| IBIS file stm32h523_533_ufbga144.ibs
[IBIS ver] 4.2
[File name] stm32h523_533_ufbga144.ibs
[File Rev] 0.2
[Date] 07-05-2024
[Source] Data Created at STMicroelectronics
[Notes]  File originated from ELDO simulations.
[Disclaimer]  This information is for modeling purpose only and is
   not guaranteed. The information is subject to change without
   notice.
[Copyright] Copyright 2024 STMicroelectronics Inc.
|   Component stm32h523_533_ufbga144
[Component] stm32h523_533_ufbga144
[Manufacturer] STMicroelectronics
[Package]
| variable   typ   min   max
R_pkg  0  NA  NA
L_pkg  0  NA  NA
C_pkg  0  NA  NA
[Pin]   signal_name   model_name
A1  VSS  gnd
A2  PB9  io8_ft_i3c_spi
A3  PB7  io8_ft_i3c_spi
A4  PB4  io8_ft_i3c_spi
A5  PG15  io8_ft_i3c_spi
A6  PG12  io8_ft_i3c_spi
A7  PG11  io8_ft_i3c_spi
A8  PD7  io8_ft_i3c_spi
A9  PD4  io8_ft_i3c_spi
A10  PD2  io8_ft_i3c_spi
A11  PC10  io8_ft_i3c_spi
A12  VSS  gnd
B1  PE2  io8_ft_i3c_spi
B2  PE0  io8_ft_i3c_spi
B3  PB8  io8_ft_i3c_spi
B4  PB6  io8_ft_i3c_spi
B5  PB3  io8_ft_i3c_spi
B6  PG14  io8_ft_i3c_spi
B7  PG10  io8_ft_i3c_spi
B8  PD6  io8_ft_i3c_spi
B9  PD3  io8_ft_i3c_spi
B10  PC12  io8_ft_i3c_spi
B11  PA14  io8_ft_i3c_spi
B12  PA10  io8_ft_i3c_spi
C1  VBAT  power
C2  PE4  io8_ft_i3c_spi
C3  PE3  io8_ft_i3c_spi
C4  BOOT0  vpphv
C5  VDDIO2  power
C6  VSS  gnd
C7  VDDIO2  power
C8  PD5  io8_ft_i3c_spi
C9  PD1  io8_ft_i3c_spi
C10  VDDUSB  power
C11  PA12  io8usb_ft_i3c_spi_phy
C12  PA11  io8usb_ft_i3c_spi_phy
D1  PC15-OSC32_OUT  io_ft_tamp
D2  PC14-OSC32_IN  io_ft_tamp
D3  PE5  io8_ft_i3c_spi
D4  VSS  gnd
D5  VCAP  nc
D6  PG13  io8_ft_i3c_spi
D7  PG9  io8_ft_i3c_spi
D8  PD0  io8_ft_i3c_spi
D9  PC11  io8_ft_i3c_spi
D10  VSS  gnd
D11  PA9  io8_ft_i3c_spi
D12  PA8  io8_ft_i3c_spi
E1  PF1  io8_ft_i3c_spi
E2  PF0  io8_ft_i3c_spi
E3  PC13  io8_ft_i3c_spi_v33
E4  PE6  io8_ft_i3c_spi
E5  VDD  power
E6  PB5  io8_ft_i3c_spi
E7  VDD  power
E8  PA15  io8_ft_i3c_spi
E9  PA13  io8_ft_i3c_spi
E10  PC9  io8_ft_i3c_spi
E11  PC8  io8_ft_i3c_spi
E12  PC7  io8_ft_i3c_spi
F1  PF5  io8_ft_i3c_spi
F2  PF4  io8_ft_i3c_spi
F3  PF3  io8_ft_i3c_spi
F4  PF2  io8_ft_i3c_spi
F5  VSS  gnd
F6  VDD  power
F7  VSS  gnd
F8  VDD  power
F9  PC6  io8_ft_i3c_spi
F10  PG8  io8_ft_i3c_spi
F11  PG7  io8_ft_i3c_spi
F12  PG6  io8_ft_i3c_spi
G1  PF6  io8_ft_i3c_spi
G2  PF7  io8_ft_i3c_spi
G3  PF9  io8_ft_i3c_spi
G4  PF8  io8_ft_i3c_spi
G5  VDD  power
G6  VSS  gnd
G7  VDD  power
G8  PD11  io8_ft_i3c_spi
G9  PD15  io8_ft_i3c_spi
G10  PG3  io8_ft_i3c_spi
G11  PG4  io8_ft_i3c_spi
G12  PG5  io8_ft_i3c_spi
H1  PH0-OSC_IN  io8_ft_i3c_spi
H2  PH1-OSC_OUT  io8_ft_i3c_spi
H3  PF10  io8_ft_i3c_spi
H4  VREFM  nc
H5  VSS  gnd
H6  VDD  power
H7  VSS  gnd
H8  PB14  nc
H9  PB15  io8_ft_spi
H10  PD12  io8_ft_i3c_spi
H11  PD14  io8_ft_i3c_spi
H12  PG2  io8_ft_i3c_spi
J1  NRST  ioreset_ft_v33
J2  PC0  io8_ft_spi
J3  VREFP  nc
J4  VDDA  nc
J5  PA7  io8_ft_spi
J6  PB1  io8_ft_spi
J7  PG1  io8_ft_i3c_spi
J8  VCAP  nc
J9  VSS  gnd
J10  PD8  io8_ft_i3c_spi
J11  PD9  io8_ft_i3c_spi
J12  PD13  io8_ft_i3c_spi
K1  PC2  io8_ft_spi
K2  PC1  io8_ft_spi
K3  VSSA  nc
K4  PA2  io8_ft_spi
K5  PC4  io8_ft_spi
K6  PB2  io8_ft_i3c_spi
K7  PF15  io8_ft_i3c_spi
K8  PE9  io8_ft_i3c_spi
K9  PE12  io8_ft_i3c_spi
K10  PE15  io8_ft_i3c_spi
K11  PB13  nc
K12  PD10  io8_ft_i3c_spi
L1  PC3  io8_ft_spi
L2  PA0  io8_ft_spi
L3  PA1  io8_ft_spi_tamp
L4  PA5  io8_ft_spi
L5  PC5  io8_ft_spi
L6  PF11  io8_ft_spi
L7  PF14  io8_ft_spi
L8  PE7  io8_ft_i3c_spi
L9  PE10  io8_ft_i3c_spi
L10  PE14  io8_ft_i3c_spi
L11  PB10  io8_ft_i3c_spi
L12  PB12  io8_ft_i3c_spi
M1  VSS  gnd
M2  PA3  io8_ft_spi
M3  PA4  io8_ft_spi
M4  PA6  io8_ft_spi
M5  PB0  io8_ft_spi
M6  PF12  io8_ft_spi
M7  PF13  io8_ft_spi
M8  PG0  io8_ft_i3c_spi
M9  PE8  io8_ft_i3c_spi
M10  PE11  io8_ft_i3c_spi
M11  PE13  io8_ft_i3c_spi
M12  VSS  gnd
[Package Model]   478-ufbga10x10-144-240126
[Pin Mapping]   pulldown_ref   pullup_ref   | Comment
A1  gndio  nc
A2  gndio  vddmmc
A3  gndio  vddio
A4  gndio  vddio
A5  gndio  vddio
A6  gndio  vddmmc
A7  gndio  vddmmc
A8  gndio  vddmmc
A9  gndio  vddio
A10  gndio  vddio
A11  gndio  vddio
A12  gndio  nc
B1  gndio  vddio
B2  gndio  vddio
B3  gndio  vddmmc
B4  gndio  vddio
B5  gndio  vddio
B6  gndio  vddmmc
B7  gndio  vddmmc
B8  gndio  vddmmc
B9  gndio  vddio
B10  gndio  vddio
B11  gndio  vddio
B12  gndio  vddio
C1  nc  vsw
C2  gndio  vddio
C3  gndio  vddio
C4  gndio  vddio
C5  nc  vddmmc
C6  gndio  nc
C7  nc  vddmmc
C8  gndio  vddio
C9  gndio  vddio
C10  nc  vddusb
C11  gndio  vddusb  | Depending on IO usage
| C11  gndio  vddio  | Depending on IO usage
C12  gndio  vddusb  | Depending on IO usage
| C12  gndio  vddio  | Depending on IO usage
D1  gndio  vddio  | Depending on IO usage
| D1  gndio  vsw  | Depending on IO usage
D2  gndio  vddio  | Depending on IO usage
| D2  gndio  vsw  | Depending on IO usage
D3  gndio  vddio
D4  gndio  nc
D5  nc  nc
D6  gndio  vddmmc
D7  gndio  vddmmc
D8  gndio  vddio
D9  gndio  vddio
D10  gndio  nc
D11  gndio  vddio
D12  gndio  vddio
E1  gndio  vddio
E2  gndio  vddio
E3  gndio  vddio  | Depending on IO usage
| E3  gndio  vsw  | Depending on IO usage
E4  gndio  vddio
E5  nc  vddio
E6  gndio  vddio
E7  nc  vddio
E8  gndio  vddio
E9  gndio  vddio
E10  gndio  vddio
E11  gndio  vddio
E12  gndio  vddio
F1  gndio  vddio
F2  gndio  vddio
F3  gndio  vddio
F4  gndio  vddio
F5  gndio  nc
F6  nc  vddio
F7  gndio  nc
F8  nc  vddio
F9  gndio  vddio
F10  gndio  vddio
F11  gndio  vddio
F12  gndio  vddio
G1  gndio  vddio
G2  gndio  vddio
G3  gndio  vddio
G4  gndio  vddio
G5  nc  vddio
G6  gndio  nc
G7  nc  vddio
G8  gndio  vddio
G9  gndio  vddio
G10  gndio  vddio
G11  gndio  vddio
G12  gndio  vddio
H1  gndio  vddio
H2  gndio  vddio
H3  gndio  vddio
H4  nc  nc
H5  gndio  nc
H6  nc  vddio
H7  gndio  nc
H8  nc  nc
H9  gndio  vddio
H10  gndio  vddio
H11  gndio  vddio
H12  gndio  vddio
J1  gndio  vddio
J2  gndio  vddio
J3  nc  nc
J4  nc  nc
J5  gndio  vddio
J6  gndio  vddio
J7  gndio  vddio
J8  nc  nc
J9  gndio  nc
J10  gndio  vddio
J11  gndio  vddio
J12  gndio  vddio
K1  gndio  vddio
K2  gndio  vddio
K3  nc  nc
K4  gndio  vddio
K5  gndio  vddio
K6  gndio  vddio
K7  gndio  vddio
K8  gndio  vddio
K9  gndio  vddio
K10  gndio  vddio
K11  nc  nc
K12  gndio  vddio
L1  gndio  vddio
L2  gndio  vddio
L3  gndio  vddio
L4  gndio  vddio
L5  gndio  vddio
L6  gndio  vddio
L7  gndio  vddio
L8  gndio  vddio
L9  gndio  vddio
L10  gndio  vddio
L11  gndio  vddio
L12  gndio  vddio
M1  gndio  nc
M2  gndio  vddio
M3  gndio  vddio
M4  gndio  vddio
M5  gndio  vddio
M6  gndio  vddio
M7  gndio  vddio
M8  gndio  vddio
M9  gndio  vddio
M10  gndio  vddio
M11  gndio  vddio
M12  gndio  nc
|[Diff Pin]  inv_pin  vdiff  tdelay_typ  tdelay_min  tdelay_max
|C11  C12  NA  NA  NA  NA
[Model Selector] io8_ft_i3c_spi
io8_ft_spi_ls_1v2 "GPIO SPI - 5V tolerant - low speed - 1.2V range"
io8_ft_spi_ls_1v8 "GPIO SPI - 5V tolerant - low speed - 1.8V range"
io8_ft_spi_ls_3v3 "GPIO SPI - 5V tolerant - low speed - 3.3V range"
io8_ft_spi_ms_1v2 "GPIO SPI - 5V tolerant - med speed - 1.2V range"
io8_ft_spi_ms_1v8 "GPIO SPI - 5V tolerant - med speed - 1.8V range"
io8_ft_spi_ms_3v3 "GPIO SPI - 5V tolerant - med speed - 3.3V range"
io8_ft_spi_fs_1v2 "GPIO SPI - 5V tolerant - fast speed - 1.2V range"
io8_ft_spi_fs_1v8 "GPIO SPI - 5V tolerant - fast speed - 1.8V range"
io8_ft_spi_fs_3v3 "GPIO SPI - 5V tolerant - fast speed - 3.3V range"
io8_ft_spi_hs_1v2 "GPIO SPI - 5V tolerant - high speed - 1.2V range"
io8_ft_spi_hs_1v8 "GPIO SPI - 5V tolerant - high speed - 1.8V range"
io8_ft_spi_hs_3v3 "GPIO SPI - 5V tolerant - high speed - 3.3V range"
io8_ft_hslv_spi_ls_1v2 "GPIO SPI low volt opt - 5V tolerant - low speed - 1.2V range"
io8_ft_hslv_spi_ls_1v8 "GPIO SPI low volt opt - 5V tolerant - low speed - 1.8V range"
io8_ft_hslv_spi_ls_2v5 "GPIO SPI low volt opt - 5V tolerant - low speed - 2.5V range"
io8_ft_hslv_spi_ms_1v2 "GPIO SPI low volt opt - 5V tolerant - med speed - 1.2V range"
io8_ft_hslv_spi_ms_1v8 "GPIO SPI low volt opt - 5V tolerant - med speed - 1.8V range"
io8_ft_hslv_spi_ms_2v5 "GPIO SPI low volt opt - 5V tolerant - med speed - 2.5V range"
io8_ft_hslv_spi_fs_1v2 "GPIO SPI low volt opt - 5V tolerant - fast speed - 1.2V range"
io8_ft_hslv_spi_fs_1v8 "GPIO SPI low volt opt - 5V tolerant - fast speed - 1.8V range"
io8_ft_hslv_spi_fs_2v5 "GPIO SPI low volt opt - 5V tolerant - fast speed - 2.5V range"
io8_ft_hslv_spi_hs_1v2 "GPIO SPI low volt opt - 5V tolerant - high speed - 1.2V range"
io8_ft_hslv_spi_hs_1v8 "GPIO SPI low volt opt - 5V tolerant - high speed - 1.8V range"
io8_ft_hslv_spi_hs_2v5 "GPIO SPI low volt opt - 5V tolerant - high speed - 2.5V range"
io8_ft_i3c_spi_ls_1v2 "GPIO SPI with I3C open-drain - 5V tolerant - low speed - 1.2V range"
io8_ft_i3c_spi_ls_1v8 "GPIO SPI with I3C open-drain - 5V tolerant - low speed - 1.8V range"
io8_ft_i3c_spi_ls_3v3 "GPIO SPI with I3C open-drain - 5V tolerant - low speed - 3.3V range"
io8_ft_i3c_spi_ms_1v2 "GPIO SPI with I3C open-drain - 5V tolerant - med speed - 1.2V range"
io8_ft_i3c_spi_ms_1v8 "GPIO SPI with I3C open-drain - 5V tolerant - med speed - 1.8V range"
io8_ft_i3c_spi_ms_3v3 "GPIO SPI with I3C open-drain - 5V tolerant - med speed - 3.3V range"
io8_ft_i3c_spi_fs_1v2 "GPIO SPI with I3C open-drain - 5V tolerant - fast speed - 1.2V range"
io8_ft_i3c_spi_fs_1v8 "GPIO SPI with I3C open-drain - 5V tolerant - fast speed - 1.8V range"
io8_ft_i3c_spi_fs_3v3 "GPIO SPI with I3C open-drain - 5V tolerant - fast speed - 3.3V range"
io8_ft_i3c_spi_hs_1v2 "GPIO SPI with I3C open-drain - 5V tolerant - high speed - 1.2V range"
io8_ft_i3c_spi_hs_1v8 "GPIO SPI with I3C open-drain - 5V tolerant - high speed - 1.8V range"
io8_ft_i3c_spi_hs_3v3 "GPIO SPI with I3C open-drain - 5V tolerant - high speed - 3.3V range"
io8_ft_hslv_i3c_spi_ls_1v2 "GPIO SPI low volt opt with I3C open-drain - 5V tolerant - low speed - 1.2V range"
io8_ft_hslv_i3c_spi_ls_1v8 "GPIO SPI low volt opt with I3C open-drain - 5V tolerant - low speed - 1.8V range"
io8_ft_hslv_i3c_spi_ls_2v5 "GPIO SPI low volt opt with I3C open-drain - 5V tolerant - low speed - 2.5V range"
io8_ft_hslv_i3c_spi_ms_1v2 "GPIO SPI low volt opt with I3C open-drain - 5V tolerant - med speed - 1.2V range"
io8_ft_hslv_i3c_spi_ms_1v8 "GPIO SPI low volt opt with I3C open-drain - 5V tolerant - med speed - 1.8V range"
io8_ft_hslv_i3c_spi_ms_2v5 "GPIO SPI low volt opt with I3C open-drain - 5V tolerant - med speed - 2.5V range"
io8_ft_hslv_i3c_spi_fs_1v2 "GPIO SPI low volt opt with I3C open-drain - 5V tolerant - fast speed - 1.2V range"
io8_ft_hslv_i3c_spi_fs_1v8 "GPIO SPI low volt opt with I3C open-drain - 5V tolerant - fast speed - 1.8V range"
io8_ft_hslv_i3c_spi_fs_2v5 "GPIO SPI low volt opt with I3C open-drain - 5V tolerant - fast speed - 2.5V range"
io8_ft_hslv_i3c_spi_hs_1v2 "GPIO SPI low volt opt with I3C open-drain - 5V tolerant - high speed - 1.2V range"
io8_ft_hslv_i3c_spi_hs_1v8 "GPIO SPI low volt opt with I3C open-drain - 5V tolerant - high speed - 1.8V range"
io8_ft_hslv_i3c_spi_hs_2v5 "GPIO SPI low volt opt with I3C open-drain - 5V tolerant - high speed - 2.5V range"
io8_ft_i3c_fmp_spi_3v3 "GPIO SPI with I3C fm+ open-drain - 5V tolerant - 3.3V range"
io8_ft_i3c_fmp_spi_1v8 "GPIO SPI with I3C fm+ open-drain - 5V tolerant - 1.8V range"
io8_ft_i3c_fmp_spi_1v2 "GPIO SPI with I3C fm+ open-drain - 5V tolerant - 1.2V range"
[Model Selector] io8_ft_i3c_spi_v33
io8_ft_spi_v33_ls_1v2 ""GPIO SPI V33 - 5V tolerant - low speed - 1.2V range"
io8_ft_spi_v33_ls_1v8 ""GPIO SPI V33 - 5V tolerant - low speed - 1.8V range"
io8_ft_spi_v33_ls_3v3 ""GPIO SPI V33 - 5V tolerant - low speed - 3.3V range"
io8_ft_spi_v33_ms_1v2 ""GPIO SPI V33 - 5V tolerant - med speed - 1.2V range"
io8_ft_spi_v33_ms_1v8 ""GPIO SPI V33 - 5V tolerant - med speed - 1.8V range"
io8_ft_spi_v33_ms_3v3 ""GPIO SPI V33 - 5V tolerant - med speed - 3.3V range"
io8_ft_spi_v33_fs_1v2 ""GPIO SPI V33 - 5V tolerant - fast speed - 1.2V range
io8_ft_spi_v33_fs_1v8 ""GPIO SPI V33 - 5V tolerant - fast speed - 1.8V range
io8_ft_spi_v33_fs_3v3 ""GPIO SPI V33 - 5V tolerant - fast speed - 3.3V range
io8_ft_spi_v33_hs_1v2 ""GPIO SPI V33 - 5V tolerant - high speed - 1.2V range
io8_ft_spi_v33_hs_1v8 ""GPIO SPI V33 - 5V tolerant - high speed - 1.8V range
io8_ft_spi_v33_hs_3v3 ""GPIO SPI V33 - 5V tolerant - high speed - 3.3V range
io8_ft_hslv_spi_v33_ls_1v2 "GPIO SPI V33 low volt opt - 5V tolerant - low speed - 1.2V range""
io8_ft_hslv_spi_v33_ls_1v8 "GPIO SPI V33 low volt opt - 5V tolerant - low speed - 1.8V range""
io8_ft_hslv_spi_v33_ls_2v5 "GPIO SPI V33 low volt opt - 5V tolerant - low speed - 2.5V range""
io8_ft_hslv_spi_v33_ms_1v2 "GPIO SPI V33 low volt opt - 5V tolerant - med speed - 1.2V range""
io8_ft_hslv_spi_v33_ms_1v8 "GPIO SPI V33 low volt opt - 5V tolerant - med speed - 1.8V range""
io8_ft_hslv_spi_v33_ms_2v5 "GPIO SPI V33 low volt opt - 5V tolerant - med speed - 2.5V range""
io8_ft_hslv_spi_v33_fs_1v2 "GPIO SPI V33 low volt opt - 5V tolerant - fast speed - 1.2V range"
io8_ft_hslv_spi_v33_fs_1v8 "GPIO SPI V33 low volt opt - 5V tolerant - fast speed - 1.8V range"
io8_ft_hslv_spi_v33_fs_2v5 "GPIO SPI V33 low volt opt - 5V tolerant - fast speed - 2.5V range"
io8_ft_hslv_spi_v33_hs_1v2 "GPIO SPI V33 low volt opt - 5V tolerant - high speed - 1.2V range"
io8_ft_hslv_spi_v33_hs_1v8 "GPIO SPI V33 low volt opt - 5V tolerant - high speed - 1.8V range"
io8_ft_hslv_spi_v33_hs_2v5 "GPIO SPI V33 low volt opt - 5V tolerant - high speed - 2.5V range"
io8_ft_i3c_spi_v33_ls_1v2 "GPIO SPI V33 with I3C open-drain - 5V tolerant - low speed - 1.2V range"
io8_ft_i3c_spi_v33_ls_1v8 "GPIO SPI V33 with I3C open-drain - 5V tolerant - low speed - 1.8V range"
io8_ft_i3c_spi_v33_ls_3v3 "GPIO SPI V33 with I3C open-drain - 5V tolerant - low speed - 3.3V range"
io8_ft_i3c_spi_v33_ms_1v2 "GPIO SPI V33 with I3C open-drain - 5V tolerant - med speed - 1.2V range"
io8_ft_i3c_spi_v33_ms_1v8 "GPIO SPI V33 with I3C open-drain - 5V tolerant - med speed - 1.8V range"
io8_ft_i3c_spi_v33_ms_3v3 "GPIO SPI V33 with I3C open-drain - 5V tolerant - med speed - 3.3V range"
io8_ft_i3c_spi_v33_fs_1v2 "GPIO SPI V33 with I3C open-drain - 5V tolerant - fast speed - 1.2V range"
io8_ft_i3c_spi_v33_fs_1v8 "GPIO SPI V33 with I3C open-drain - 5V tolerant - fast speed - 1.8V range"
io8_ft_i3c_spi_v33_fs_3v3 "GPIO SPI V33 with I3C open-drain - 5V tolerant - fast speed - 3.3V range"
io8_ft_i3c_spi_v33_hs_1v2 "GPIO SPI V33 with I3C open-drain - 5V tolerant - high speed - 1.2V range"
io8_ft_i3c_spi_v33_hs_1v8 "GPIO SPI V33 with I3C open-drain - 5V tolerant - high speed - 1.8V range"
io8_ft_i3c_spi_v33_hs_3v3 "GPIO SPI V33 with I3C open-drain - 5V tolerant - high speed - 3.3V range"
io8_ft_hslv_i3c_spi_v33_ls_1v2 "GPIO SPI V33 low volt opt with I3C open-drain - 5V tolerant - low speed - 1.2V range"
io8_ft_hslv_i3c_spi_v33_ls_1v8 "GPIO SPI V33 low volt opt with I3C open-drain - 5V tolerant - low speed - 1.8V range"
io8_ft_hslv_i3c_spi_v33_ls_2v5 "GPIO SPI V33 low volt opt with I3C open-drain - 5V tolerant - low speed - 2.5V range"
io8_ft_hslv_i3c_spi_v33_ms_1v2 "GPIO SPI V33 low volt opt with I3C open-drain - 5V tolerant - med speed - 1.2V range"
io8_ft_hslv_i3c_spi_v33_ms_1v8 "GPIO SPI V33 low volt opt with I3C open-drain - 5V tolerant - med speed - 1.8V range"
io8_ft_hslv_i3c_spi_v33_ms_2v5 "GPIO SPI V33 low volt opt with I3C open-drain - 5V tolerant - med speed - 2.5V range"
io8_ft_hslv_i3c_spi_v33_fs_1v2 "GPIO SPI V33 low volt opt with I3C open-drain - 5V tolerant - fast speed - 1.2V range"
io8_ft_hslv_i3c_spi_v33_fs_1v8 "GPIO SPI V33 low volt opt with I3C open-drain - 5V tolerant - fast speed - 1.8V range"
io8_ft_hslv_i3c_spi_v33_fs_2v5 "GPIO SPI V33 low volt opt with I3C open-drain - 5V tolerant - fast speed - 2.5V range"
io8_ft_hslv_i3c_spi_v33_hs_1v2 "GPIO SPI V33 low volt opt with I3C open-drain - 5V tolerant - high speed - 1.2V range"
io8_ft_hslv_i3c_spi_v33_hs_1v8 "GPIO SPI V33 low volt opt with I3C open-drain - 5V tolerant - high speed - 1.8V range"
io8_ft_hslv_i3c_spi_v33_hs_2v5 "GPIO SPI V33 low volt opt with I3C open-drain - 5V tolerant - high speed - 2.5V range"
io8_ft_i3c_fmp_spi_v33_3v3 "GPIO SPI V33 with I3C fm+ open-drain - 5V tolerant - 3.3V range"
io8_ft_i3c_fmp_spi_v33_1v8 "GPIO SPI V33 with I3C fm+ open-drain - 5V tolerant - 1.8V range"
io8_ft_i3c_fmp_spi_v33_1v2 "GPIO SPI V33 with I3C fm+ open-drain - 5V tolerant - 1.2V range"
[Model Selector] io8_ft_spi
io8_ft_spi_ls_1v2 "GPIO SPI - 5V tolerant - low speed - 1.2V range"
io8_ft_spi_ls_1v8 "GPIO SPI - 5V tolerant - low speed - 1.8V range"
io8_ft_spi_ls_3v3 "GPIO SPI - 5V tolerant - low speed - 3.3V range"
io8_ft_spi_ms_1v2 "GPIO SPI- 5V tolerant - med speed - 1.2V range"
io8_ft_spi_ms_1v8 "GPIO SPI- 5V tolerant - med speed - 1.8V range"
io8_ft_spi_ms_3v3 "GPIO SPI- 5V tolerant - med speed - 3.3V range"
io8_ft_spi_fs_1v2 "GPIO SPI- 5V tolerant - fast speed - 1.2V range"
io8_ft_spi_fs_1v8 "GPIO SPI- 5V tolerant - fast speed - 1.8V range"
io8_ft_spi_fs_3v3 "GPIO SPI- 5V tolerant - fast speed - 3.3V range"
io8_ft_spi_hs_1v2 "GPIO SPI- 5V tolerant - high speed - 1.2V range"
io8_ft_spi_hs_1v8 "GPIO SPI- 5V tolerant - high speed - 1.8V range"
io8_ft_spi_hs_3v3 "GPIO SPI- 5V tolerant - high speed - 3.3V range"
io8_ft_hslv_spi_ls_1v2 "GPIO SPI low volt opt - 5V tolerant - low speed - 1.2V range"
io8_ft_hslv_spi_ls_1v8 "GPIO SPI low volt opt - 5V tolerant - low speed - 1.8V range"
io8_ft_hslv_spi_ls_2v5 "GPIO SPI low volt opt - 5V tolerant - low speed - 2.5V range"
io8_ft_hslv_spi_ms_1v2 "GPIO SPI low volt opt - 5V tolerant - med speed - 1.2V range"
io8_ft_hslv_spi_ms_1v8 "GPIO SPI low volt opt - 5V tolerant - med speed - 1.8V range"
io8_ft_hslv_spi_ms_2v5 "GPIO SPI low volt opt - 5V tolerant - med speed - 2.5V range"
io8_ft_hslv_spi_fs_1v2 "GPIO SPI low volt opt - 5V tolerant - fast speed - 1.2V range"
io8_ft_hslv_spi_fs_1v8 "GPIO SPI low volt opt - 5V tolerant - fast speed - 1.8V range"
io8_ft_hslv_spi_fs_2v5 "GPIO SPI low volt opt - 5V tolerant - fast speed - 2.5V range"
io8_ft_hslv_spi_hs_1v2 "GPIO SPI low volt opt - 5V tolerant - high speed - 1.2V range"
io8_ft_hslv_spi_hs_1v8 "GPIO SPI low volt opt - 5V tolerant - high speed - 1.8V range"
io8_ft_hslv_spi_hs_2v5 "GPIO SPI low volt opt - 5V tolerant - high speed - 2.5V range"
[Model Selector] io8_ft_spi_tamp
io8_ft_spi_ls_1v2 "GPIO SPI - 5V tolerant - low speed - 1.2V range"
io8_ft_spi_ls_1v8 "GPIO SPI - 5V tolerant - low speed - 1.8V range"
io8_ft_spi_ls_3v3 "GPIO SPI- 5V tolerant - low speed - 3.3V range"
io8_ft_spi_ms_1v2 "GPIO SPI - 5V tolerant - med speed - 1.2V range"
io8_ft_spi_ms_1v8 "GPIO SPI - 5V tolerant - med speed - 1.8V range"
io8_ft_spi_ms_3v3 "GPIO SPI - 5V tolerant - med speed - 3.3V range"
io8_ft_spi_fs_1v2 "GPIO SPI - 5V tolerant - fast speed - 1.2V range"
io8_ft_spi_fs_1v8 "GPIO SPI - 5V tolerant - fast speed - 1.8V range"
io8_ft_spi_fs_3v3 "GPIO SPI - 5V tolerant - fast speed - 3.3V range"
io8_ft_spi_hs_1v2 "GPIO SPI - 5V tolerant - high speed - 1.2V range"
io8_ft_spi_hs_1v8 "GPIO SPI - 5V tolerant - high speed - 1.8V range"
io8_ft_spi_hs_3v3 "GPIO SPI - 5V tolerant - high speed - 3.3V range"
io8_ft_hslv_spi_ls_1v2 "GPIO SPI low volt opt - 5V tolerant - low speed - 1.2V range"
io8_ft_hslv_spi_ls_1v8 "GPIO SPI low volt opt - 5V tolerant - low speed - 1.8V range"
io8_ft_hslv_spi_ls_2v5 "GPIO SPI low volt opt - 5V tolerant - low speed - 2.5V range"
io8_ft_hslv_spi_ms_1v2 "GPIO SPI low volt opt - 5V tolerant - med speed - 1.2V range"
io8_ft_hslv_spi_ms_1v8 "GPIO SPI low volt opt - 5V tolerant - med speed - 1.8V range"
io8_ft_hslv_spi_ms_2v5 "GPIO SPI low volt opt - 5V tolerant - med speed - 2.5V range"
io8_ft_hslv_spi_fs_1v2 "GPIO SPI low volt opt - 5V tolerant - fast speed - 1.2V range"
io8_ft_hslv_spi_fs_1v8 "GPIO SPI low volt opt - 5V tolerant - fast speed - 1.8V range"
io8_ft_hslv_spi_fs_2v5 "GPIO SPI low volt opt - 5V tolerant - fast speed - 2.5V range"
io8_ft_hslv_spi_hs_1v2 "GPIO SPI low volt opt - 5V tolerant - high speed - 1.2V range"
io8_ft_hslv_spi_hs_1v8 "GPIO SPI low volt opt - 5V tolerant - high speed - 1.8V range"
io8_ft_hslv_spi_hs_2v5 "GPIO SPI low volt opt - 5V tolerant - high speed - 2.5V range
io8_ft_tamp_v33_1v2 "IO tamper - 5V tolerant - 1.2V range"
io8_ft_tamp_v33_1v8 "IO tamper - 5V tolerant - 1.8V range"
io8_ft_tamp_v33_3v3 "IO tamper - 5V tolerant - 3.3V range"
[Model Selector] io8usb_ft_i3c_spi_phy
io8_ft_spi_ls_1v2 "GPIO SPI - 5V tolerant - low speed - 1.2V range"
io8_ft_spi_ls_1v8 "GPIO SPI - 5V tolerant - low speed - 1.8V range"
io8_ft_spi_ls_3v3 "GPIO SPI - 5V tolerant - low speed - 3.3V range"
io8_ft_spi_ms_1v2 "GPIO SPI - 5V tolerant - med speed - 1.2V range"
io8_ft_spi_ms_1v8 "GPIO SPI - 5V tolerant - med speed - 1.8V range"
io8_ft_spi_ms_3v3 "GPIO SPI - 5V tolerant - med speed - 3.3V range"
io8_ft_spi_fs_1v2 "GPIO SPI - 5V tolerant - fast speed - 1.2V range"
io8_ft_spi_fs_1v8 "GPIO SPI - 5V tolerant - fast speed - 1.8V range"
io8_ft_spi_fs_3v3 "GPIO SPI - 5V tolerant - fast speed - 3.3V range"
io8_ft_spi_hs_1v2 "GPIO SPI - 5V tolerant - high speed - 1.2V range"
io8_ft_spi_hs_1v8 "GPIO SPI - 5V tolerant - high speed - 1.8V range"
io8_ft_spi_hs_3v3 "GPIO SPI - 5V tolerant - high speed - 3.3V range"
io8_ft_hslv_spi_ls_1v2 "GPIO SPI low volt opt - 5V tolerant - low speed - 1.2V range"
io8_ft_hslv_spi_ls_1v8 "GPIO SPI low volt opt - 5V tolerant - low speed - 1.8V range"
io8_ft_hslv_spi_ls_2v5 "GPIO SPI low volt opt - 5V tolerant - low speed - 2.5V range"
io8_ft_hslv_spi_ms_1v2 "GPIO SPI low volt opt - 5V tolerant - med speed - 1.2V range"
io8_ft_hslv_spi_ms_1v8 "GPIO SPI low volt opt - 5V tolerant - med speed - 1.8V range"
io8_ft_hslv_spi_ms_2v5 "GPIO SPI low volt opt - 5V tolerant - med speed - 2.5V range"
io8_ft_hslv_spi_fs_1v2 "GPIO SPI low volt opt - 5V tolerant - fast speed - 1.2V range"
io8_ft_hslv_spi_fs_1v8 "GPIO SPI low volt opt - 5V tolerant - fast speed - 1.8V range"
io8_ft_hslv_spi_fs_2v5 "GPIO SPI low volt opt - 5V tolerant - fast speed - 2.5V range"
io8_ft_hslv_spi_hs_1v2 "GPIO SPI low volt opt - 5V tolerant - high speed - 1.2V range"
io8_ft_hslv_spi_hs_1v8 "GPIO SPI low volt opt - 5V tolerant - high speed - 1.8V range"
io8_ft_hslv_spi_hs_2v5 "GPIO SPI low volt opt - 5V tolerant - high speed - 2.5V range"
io8_ft_i3c_spi_ls_1v2 "GPIO SPI  with I3C open-drain - 5V tolerant - low speed - 1.2V range"
io8_ft_i3c_spi_ls_1v8 "GPIO SPI  with I3C open-drain - 5V tolerant - low speed - 1.8V range"
io8_ft_i3c_spi_ls_3v3 "GPIO SPI  with I3C open-drain - 5V tolerant - low speed - 3.3V range"
io8_ft_i3c_spi_ms_1v2 "GPIO SPI  with I3C open-drain - 5V tolerant - med speed - 1.2V range"
io8_ft_i3c_spi_ms_1v8 "GPIO SPI  with I3C open-drain - 5V tolerant - med speed - 1.8V range"
io8_ft_i3c_spi_ms_3v3 "GPIO SPI  with I3C open-drain - 5V tolerant - med speed - 3.3V range"
io8_ft_i3c_spi_fs_1v2 "GPIO SPI  with I3C open-drain - 5V tolerant - fast speed - 1.2V range"
io8_ft_i3c_spi_fs_1v8 "GPIO SPI  with I3C open-drain - 5V tolerant - fast speed - 1.8V range"
io8_ft_i3c_spi_fs_3v3 "GPIO SPI  with I3C open-drain - 5V tolerant - fast speed - 3.3V range"
io8_ft_i3c_spi_hs_1v2 "GPIO SPI  with I3C open-drain - 5V tolerant - high speed - 1.2V range"
io8_ft_i3c_spi_hs_1v8 "GPIO SPI  with I3C open-drain - 5V tolerant - high speed - 1.8V range"
io8_ft_i3c_spi_hs_3v3 "GPIO SPI  with I3C open-drain - 5V tolerant - high speed - 3.3V range"
io8_ft_hslv_i3c_spi_ls_1v2 "GPIO SPI  low volt opt with I3C open-drain - 5V tolerant - low speed - 1.2V range"
io8_ft_hslv_i3c_spi_ls_1v8 "GPIO SPI  low volt opt with I3C open-drain - 5V tolerant - low speed - 1.8V range"
io8_ft_hslv_i3c_spi_ls_2v5 "GPIO SPI  low volt opt with I3C open-drain - 5V tolerant - low speed - 2.5V range"
io8_ft_hslv_i3c_spi_ms_1v2 "GPIO SPI  low volt opt with I3C open-drain - 5V tolerant - med speed - 1.2V range"
io8_ft_hslv_i3c_spi_ms_1v8 "GPIO SPI  low volt opt with I3C open-drain - 5V tolerant - med speed - 1.8V range"
io8_ft_hslv_i3c_spi_ms_2v5 "GPIO SPI  low volt opt with I3C open-drain - 5V tolerant - med speed - 2.5V range"
io8_ft_hslv_i3c_spi_fs_1v2 "GPIO SPI  low volt opt with I3C open-drain - 5V tolerant - fast speed - 1.2V range"
io8_ft_hslv_i3c_spi_fs_1v8 "GPIO SPI  low volt opt with I3C open-drain - 5V tolerant - fast speed - 1.8V range"
io8_ft_hslv_i3c_spi_fs_2v5 "GPIO SPI  low volt opt with I3C open-drain - 5V tolerant - fast speed - 2.5V range"
io8_ft_hslv_i3c_spi_hs_1v2 "GPIO SPI  low volt opt with I3C open-drain - 5V tolerant - high speed - 1.2V range"
io8_ft_hslv_i3c_spi_hs_1v8 "GPIO SPI  low volt opt with I3C open-drain - 5V tolerant - high speed - 1.8V range"
io8_ft_hslv_i3c_spi_hs_2v5 "GPIO SPI  low volt opt with I3C open-drain - 5V tolerant - high speed - 2.5V range"
io8_ft_i3c_fmp_spi_3v3 "GPIO SPI  with I3C fm+ open-drain - 5V tolerant - 3.3V range"
io8_ft_i3c_fmp_spi_1v8 "GPIO SPI  with I3C fm+ open-drain - 5V tolerant - 1.8V range"
io8_ft_i3c_fmp_spi_1v2 "GPIO SPI  with I3C fm+ open-drain - 5V tolerant - 1.2V range"
io8usb_ft_phy_ls_2v5 "USB PHY - 5V tolerant - low speed - 2.5V range"
io8usb_ft_phy_ls_3v3 "USB PHY - 5V tolerant - low speed - 3.3V range
io8usb_ft_phy_fs_2v5 "USB PHY - 5V tolerant - fast speed - 2.5V range"
io8usb_ft_phy_fs_3v3 "USB PHY - 5V tolerant - fast speed - 3.3V range"
[Model Selector] io_ft_tamp
io_ft_tamp_3v3 "IO tamper - 5V tolerant - 3.3V range"
io_ft_tamp_1v8 "IO tamper - 5V tolerant - 1.8V range"
io_ft_tamp_1v2 "IO tamper - 5V tolerant - 1.2V range"
[Model Selector] ioreset_ft_v33
ioreset_ft_v33_1v2 "Reset PAD. 5V tolerant. 1.2V range"
ioreset_ft_v33_1v8 "Reset PAD. 5V tolerant. 1.8V range"
ioreset_ft_v33_3v3 "Reset PAD. 5V tolerant. 3.3V range"
[Model Selector] vpphv
vpphv_1v2 "Flash Test cell v33 = 1.2 V range"
vpphv_1v8 "Flash Test cell v33 = 1.8 V range"
vpphv_3v3 "Flash Test cell v33 = 3.3 V range"
[Define Package Model]  478-ufbga10x10-144-240126
[Manufacturer]  unknown
[OEM]  unknown
[Description]  unknown
[Number Of Pins]  125
[Pin Numbers]
| Pin Name Terminal   Net Name   Starting Node   Ending Node
C4 | BOOT0
J1 | NRST
L2 | PA0
L3 | PA1
K4 | PA2
M2 | PA3
M3 | PA4
L4 | PA5
M4 | PA6
J5 | PA7
D12 | PA8
D11 | PA9
B12 | PA10
C12 | PA11
C11 | PA12
E9 | PA13
B11 | PA14
E8 | PA15
M5 | PB0
J6 | PB1
K6 | PB2
B5 | PB3
A4 | PB4
E6 | PB5
B4 | PB6
A3 | PB7
B3 | PB8
A2 | PB9
L11 | PB10
L12 | PB12
K11 | PB13
H8 | PB14
H9 | PB15
J2 | PC0
K2 | PC1
K1 | PC2
L1 | PC3
K5 | PC4
L5 | PC5
F9 | PC6
E12 | PC7
E11 | PC8
E10 | PC9
A11 | PC10
D9 | PC11
B10 | PC12
E3 | PC13
D2 | PC14-OSC32_IN
D1 | PC15-OSC32_OUT
D8 | PD0
C9 | PD1
A10 | PD2
B9 | PD3
A9 | PD4
C8 | PD5
B8 | PD6
A8 | PD7
J10 | PD8
J11 | PD9
K12 | PD10
G8 | PD11
H10 | PD12
J12 | PD13
H11 | PD14
G9 | PD15
B2 | PE0
B1 | PE2
C3 | PE3
C2 | PE4
D3 | PE5
E4 | PE6
L8 | PE7
M9 | PE8
K8 | PE9
L9 | PE10
M10 | PE11
K9 | PE12
M11 | PE13
L10 | PE14
K10 | PE15
E2 | PF0
E1 | PF1
F4 | PF2
F3 | PF3
F2 | PF4
F1 | PF5
G1 | PF6
G2 | PF7
G4 | PF8
G3 | PF9
H3 | PF10
L6 | PF11
M6 | PF12
M7 | PF13
L7 | PF14
K7 | PF15
M8 | PG0
J7 | PG1
H12 | PG2
G10 | PG3
G11 | PG4
G12 | PG5
F12 | PG6
F11 | PG7
F10 | PG8
D7 | PG9
B7 | PG10
A7 | PG11
A6 | PG12
D6 | PG13
B6 | PG14
A5 | PG15
H1 | PH0-OSC_IN
H2 | PH1-OSC_OUT
C1 | VBAT
J8 | VCAP
D5 | VCAP
E5 | VDD
J4 | VDDA
C5 | VDDIO2
C10 | VDDUSB
H4 | VREFM
J3 | VREFP
A1 | VSS
K3 | VSSA
|[Merged Pins]  E5
|E7  |  VDD
|F6  |  VDD
|F8  |  VDD
|G5  |  VDD
|G7  |  VDD
|H6  |  VDD
|[Merged Pins]  C5
|C7  |  VDDIO2
|[Merged Pins]  A1
|A12  |  VSS
|C6  |  VSS
|D4  |  VSS
|D10  |  VSS
|F5  |  VSS
|F7  |  VSS
|G6  |  VSS
|H5  |  VSS
|H7  |  VSS
|J9  |  VSS
|M1  |  VSS
|M12  |  VSS
[Model Data]
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[End Model Data]
[End Package Model]
|End [Component]
| Models and submodels in the file (118): io8_ft_hslv_i3c_spi_fs_1v2 (I/O_open_drain), io8_ft_hslv_i3c_spi_fs_1v8 (I/O_open_drain), io8_ft_hslv_i3c_spi_fs_2v5 (I/O_open_drain), io8_ft_hslv_i3c_spi_hs_1v2 (I/O_open_drain), io8_ft_hslv_i3c_spi_hs_1v8 (I/O_open_drain), io8_ft_hslv_i3c_spi_hs_2v5 (I/O_open_drain), io8_ft_hslv_i3c_spi_ls_1v2 (I/O_open_drain), io8_ft_hslv_i3c_spi_ls_1v8 (I/O_open_drain), io8_ft_hslv_i3c_spi_ls_2v5 (I/O_open_drain), io8_ft_hslv_i3c_spi_ms_1v2 (I/O_open_drain), io8_ft_hslv_i3c_spi_ms_1v8 (I/O_open_drain), io8_ft_hslv_i3c_spi_ms_2v5 (I/O_open_drain), io8_ft_hslv_i3c_spi_v33_fs_1v2 (I/O_open_drain), io8_ft_hslv_i3c_spi_v33_fs_1v8 (I/O_open_drain), io8_ft_hslv_i3c_spi_v33_fs_2v5 (I/O_open_drain), io8_ft_hslv_i3c_spi_v33_hs_1v2 (I/O_open_drain), io8_ft_hslv_i3c_spi_v33_hs_1v8 (I/O_open_drain), io8_ft_hslv_i3c_spi_v33_hs_2v5 (I/O_open_drain), io8_ft_hslv_i3c_spi_v33_ls_1v2 (I/O_open_drain), io8_ft_hslv_i3c_spi_v33_ls_1v8 (I/O_open_drain), io8_ft_hslv_i3c_spi_v33_ls_2v5 (I/O_open_drain), io8_ft_hslv_i3c_spi_v33_ms_1v2 (I/O_open_drain), io8_ft_hslv_i3c_spi_v33_ms_1v8 (I/O_open_drain), io8_ft_hslv_i3c_spi_v33_ms_2v5 (I/O_open_drain), io8_ft_hslv_spi_fs_1v2 (I/O), io8_ft_hslv_spi_fs_1v8 (I/O), io8_ft_hslv_spi_fs_2v5 (I/O), io8_ft_hslv_spi_hs_1v2 (I/O), io8_ft_hslv_spi_hs_1v8 (I/O), io8_ft_hslv_spi_hs_2v5 (I/O), io8_ft_hslv_spi_ls_1v2 (I/O), io8_ft_hslv_spi_ls_1v8 (I/O), io8_ft_hslv_spi_ls_2v5 (I/O), io8_ft_hslv_spi_ms_1v2 (I/O), io8_ft_hslv_spi_ms_1v8 (I/O), io8_ft_hslv_spi_ms_2v5 (I/O), io8_ft_hslv_spi_v33_fs_1v2 (I/O), io8_ft_hslv_spi_v33_fs_1v8 (I/O), io8_ft_hslv_spi_v33_fs_2v5 (I/O), io8_ft_hslv_spi_v33_hs_1v2 (I/O), io8_ft_hslv_spi_v33_hs_1v8 (I/O), io8_ft_hslv_spi_v33_hs_2v5 (I/O), io8_ft_hslv_spi_v33_ls_1v2 (I/O), io8_ft_hslv_spi_v33_ls_1v8 (I/O), io8_ft_hslv_spi_v33_ls_2v5 (I/O), io8_ft_hslv_spi_v33_ms_1v2 (I/O), io8_ft_hslv_spi_v33_ms_1v8 (I/O), io8_ft_hslv_spi_v33_ms_2v5 (I/O), io8_ft_i3c_fmp_spi_1v2 (I/O_open_drain), io8_ft_i3c_fmp_spi_1v8 (I/O_open_drain), io8_ft_i3c_fmp_spi_3v3 (I/O_open_drain), io8_ft_i3c_fmp_spi_v33_1v2 (I/O_open_drain), io8_ft_i3c_fmp_spi_v33_1v8 (I/O_open_drain), io8_ft_i3c_fmp_spi_v33_3v3 (I/O_open_drain), io8_ft_i3c_spi_fs_1v2 (I/O_open_drain), io8_ft_i3c_spi_fs_1v8 (I/O_open_drain), io8_ft_i3c_spi_fs_3v3 (I/O_open_drain), io8_ft_i3c_spi_hs_1v2 (I/O_open_drain), io8_ft_i3c_spi_hs_1v8 (I/O_open_drain), io8_ft_i3c_spi_hs_3v3 (I/O_open_drain), io8_ft_i3c_spi_ls_1v2 (I/O_open_drain), io8_ft_i3c_spi_ls_1v8 (I/O_open_drain), io8_ft_i3c_spi_ls_3v3 (I/O_open_drain), io8_ft_i3c_spi_ms_1v2 (I/O_open_drain), io8_ft_i3c_spi_ms_1v8 (I/O_open_drain), io8_ft_i3c_spi_ms_3v3 (I/O_open_drain), io8_ft_i3c_spi_v33_fs_1v2 (I/O_open_drain), io8_ft_i3c_spi_v33_fs_1v8 (I/O_open_drain), io8_ft_i3c_spi_v33_fs_3v3 (I/O_open_drain), io8_ft_i3c_spi_v33_hs_1v2 (I/O_open_drain), io8_ft_i3c_spi_v33_hs_1v8 (I/O_open_drain), io8_ft_i3c_spi_v33_hs_3v3 (I/O_open_drain), io8_ft_i3c_spi_v33_ls_1v2 (I/O_open_drain), io8_ft_i3c_spi_v33_ls_1v8 (I/O_open_drain), io8_ft_i3c_spi_v33_ls_3v3 (I/O_open_drain), io8_ft_i3c_spi_v33_ms_1v2 (I/O_open_drain), io8_ft_i3c_spi_v33_ms_1v8 (I/O_open_drain), io8_ft_i3c_spi_v33_ms_3v3 (I/O_open_drain), io8_ft_spi_fs_1v2 (I/O), io8_ft_spi_fs_1v8 (I/O)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
